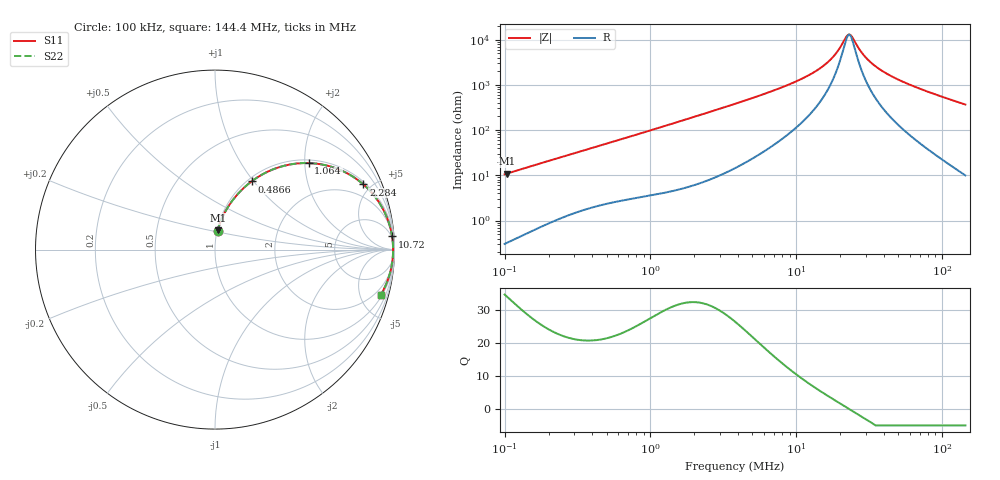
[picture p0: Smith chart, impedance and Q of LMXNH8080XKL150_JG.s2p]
! LMXNH8080XKL150_JG  S-PARAMETER MODEL  ( General Type )
! Model Generated by TAIYO YUDEN Corporation (http://www.ty-top.com)
! Version 1.0
! TAIYO YUDEN Control No. 191025NI43SB-FBB
! Copyright(c) 2019 TAIYO YUDEN CO.,LTD. All Rights Reserved.
! Product Description (link to TY-COMPAS)
! https://ds.yuden.co.jp/TYCOMPAS/or/detail?pn=LMXNH8080XKL150MJG&u=M
! Products Name : Inductors
! Characteristics :
!  Inductance : 15 uH , SRF(min) : 20 MHz , DC Resistance(max) : 0.078 Ohm
!  Rated Current : Saturation :2000 mA , Temp Rise : 2200 mA
!  Case Size : 8.0 x 8.0 / 0.315 x 0.315 [mm/inch] , Thickness : 3 / 0.118 [mm/inch]
!  (Conditions: Temperature = 25 degC , DC Bias Current/Voltage = 0A / 0V)
! External Node Assignments :
!  1  o---GGG---o  2
! GND o---------o GND
! Frequency Range : 0.1MHz  -  144.390904MHz  [ 402 STEP ]
# MHz S RI R 50
! Freq[MHz].  S11 Real  S11 Imag  S21 Real  S21 Imag  S12 Real  S12 Imag  S22 Real  S22 Imag
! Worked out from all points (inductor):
!   401 points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, 100 kHz to 144.4 MHz, reference 50 ohm
!   read as one part in series: L = 16.7 uH near 103.7 kHz
!   highest Q = 33.9 at 103.7 kHz (marker M1), where L = 16.8 uH
!   self-resonance near 23 MHz
!   S11 on the Smith chart (normalised r, x): 100 kHz: 1.01, +0.21; 486.6 kHz: 1.05, +0.98; 1.064 MHz: 1.07, +2.09; 2.284 MHz: 1.14, +4.49; 10.72 MHz: 4, +26; 144.4 MHz: 1.20, -7.33
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0.1  0.014 0.1037  0.986 -0.1037  0.986 -0.1037  0.014 0.1037
0.103705  0.0149 0.1074  0.9851 -0.1074  0.9851 -0.1074  0.0149 0.1074
0.338238  0.1177 0.299  0.8823 -0.299  0.8823 -0.299  0.1177 0.299
0.486631  0.2037 0.3799  0.7963 -0.3799  0.7963 -0.3799  0.2037 0.3799
0.752961  0.3625 0.4607  0.6375 -0.4607  0.6375 -0.4607  0.3625 0.4607
1.063777  0.5218 0.4821  0.4782 -0.4821  0.4782 -0.4821  0.5218 0.4821
1.144052  0.5564 0.4798  0.4436 -0.4798  0.4436 -0.4798  0.5564 0.4798
2.283506  0.8271 0.3628  0.1729 -0.3628  0.1729 -0.3628  0.8271 0.3628
3.869624  0.9296 0.2375  0.0704 -0.2375  0.0704 -0.2375  0.9296 0.2375
6.925194  0.9742 0.1304  0.0258 -0.1304  0.0258 -0.1304  0.9742 0.1304
10.7153  0.9866 0.0736  0.0134 -0.0736  0.0134 -0.0736  0.9866 0.0736
12.85266  0.9892 0.0541  0.0108 -0.0541  0.0108 -0.0541  0.9892 0.0541
17.1939  0.9916 0.0261  0.0084 -0.0261  0.0084 -0.0261  0.9916 0.0261
19.17642  0.992 0.0162  0.00796 -0.0162  0.00796 -0.0162  0.992 0.0162
21.78008  0.9923 0.00494  0.0077 -0.00494  0.0077 -0.00494  0.9923 0.00494
23.00149  0.9923 0.000143  0.00766 -0.000143  0.00766 -0.000143  0.9923 0.000143
24.2914  0.9923 -0.00465  0.00768 0.00465  0.00768 0.00465  0.9923 -0.00465
27.58954  0.9921 -0.0159  0.00789 0.0159  0.00789 0.0159  0.9921 -0.0159
31.33549  0.9916 -0.0274  0.00838 0.0274  0.00838 0.0274  0.9916 -0.0274
43.47261  0.9888 -0.0594  0.0112 0.0594  0.0112 0.0594  0.9888 -0.0594
71.03701  0.9779 -0.1195  0.0221 0.1195  0.0221 0.1195  0.9779 -0.1195
144.3909  0.9249 -0.2504  0.0751 0.2504  0.0751 0.2504  0.9249 -0.2504
